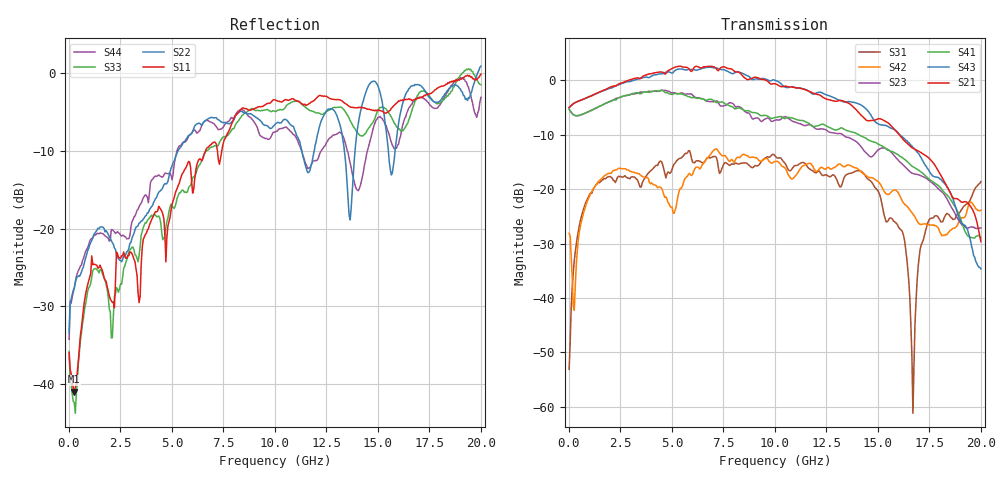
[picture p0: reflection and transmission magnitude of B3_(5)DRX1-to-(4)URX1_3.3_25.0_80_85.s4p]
!Agilent Technologies,N5225A,MY51451112,A.09.50.13
!Agilent N5225A: A.09.50.13
!Date: Sunday, March 12, 2017 05:21:35
!Correction: S11(Full 4 Port(1,2,3,4))
!S12(Full 4 Port(1,2,3,4))
!S13(Full 4 Port(1,2,3,4))
!S14(Full 4 Port(1,2,3,4))
!S21(Full 4 Port(1,2,3,4))
!S22(Full 4 Port(1,2,3,4))
!S23(Full 4 Port(1,2,3,4))
!S24(Full 4 Port(1,2,3,4))
!S31(Full 4 Port(1,2,3,4))
!S32(Full 4 Port(1,2,3,4))
!S33(Full 4 Port(1,2,3,4))
!S34(Full 4 Port(1,2,3,4))
!S41(Full 4 Port(1,2,3,4))
!S42(Full 4 Port(1,2,3,4))
!S43(Full 4 Port(1,2,3,4))
!S44(Full 4 Port(1,2,3,4))
!S4P File: Measurements: <S11,S12,S13,S14>,
!<S21,S22,S23,S24>,
!<S31,S32,S33,S34>,
!<S41,S42,S43,S44>:
# Hz S  dB  R 50
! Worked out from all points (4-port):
!   401 points, 10 MHz to 20 GHz, reference 50 ohm
!   strongest paths, dB at 10 MHz, 5.008 GHz, 10.01 GHz, 15 GHz, 20 GHz:
!     S21: -5.0, 2.2, -0.7, -7.1, -29.6
!     S43: -5.0, 1.3, 0.0, -8.0, -34.7
!     S41: -5.3, -2.6, -6.9, -11.7, -28.9
!     S23: -5.3, -2.3, -7.3, -12.8, -27.1
!     S42: -28.1, -23.3, -14.9, -18.6, -23.9
!     S31: -53.1, -16.4, -13.9, -20.3, -18.6
!   lowest |S11| = -40.9 dB at 259.9 MHz (marker M1), VSWR 1.02, Z = 50.3 - j0.86 ohm
!   |S11| at or under -10 dB: start of sweep to 6.636 GHz; 7.207 GHz to 7.422 GHz (214.9 MHz wide, 2.94 % of centre)
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1e7  -35.94 -38.5  -66.81 145.0  -53.30 11.9  -77.60 160.5
     -5.02 1.4  -33.41 38.9  -5.33 -179.9  -28.03 37.7
     -53.11 17.5  -71.79 97.3  -35.75 -45.8  -64.70 94.1
     -5.33 -179.9  -28.10 38.0  -5.00 1.6  -34.23 44.1
2.59875e8  -40.92 -72.0  -49.86 56.0  -33.16 94.7  -50.74 54.6
           -4.21 -2.2  -27.63 -131.8  -6.43 169.7  -41.81 -161.8
           -33.21 95.3  -49.91 57.8  -42.28 -78.8  -50.44 56.6
           -6.43 168.9  -42.26 -171.1  -4.19 -3.0  -27.67 -137.7
5.157425e9  -15.53 88.5  -37.75 12.0  -15.42 29.2  -39.42 -18.5
            2.41 173.7  -10.99 143.9  -2.36 -27.1  -24.24 57.7
            -15.21 27.6  -37.57 1.9  -17.15 103.9  -38.59 -54.3
            -2.43 -42.8  -23.82 59.0  1.80 163.8  -11.01 122.8
8.255875e9  -5.04 37.1  -39.67 -109.5  -15.53 -0.5  -36.36 -138.8
            1.46 21.1  -5.06 80.8  -4.85 -161.1  -13.85 47.6
            -15.39 -1.1  -32.44 -115.7  -6.08 58.7  -31.73 -151.8
            -5.06 175.9  -14.21 50.2  1.48 8.3  -4.87 45.5
1.215392e10  -2.93 -17.6  -33.33 -149.2  -16.32 -21.1  -34.60 170.5
             -2.69 -145.1  -7.01 66.9  -8.99 37.4  -16.04 40.2
             -16.68 -20.3  -34.12 -142.1  -5.20 -3.6  -33.11 175.4
             -8.29 1.3  -16.29 42.9  -2.19 -169.3  -10.57 -6.3
1.670165e10  -3.53 -75.7  -34.84 118.1  -50.91 9.9  -36.57 86.3
             -12.49 13.7  -1.63 65.9  -17.14 170.5  -24.78 57.1
             -61.18 55.9  -33.11 122.1  -4.42 -82.3  -33.10 84.0
             -15.88 118.3  -24.62 57.3  -12.32 -36.2  -3.70 -61.2
2e10  -0.18 -114.1  -32.97 63.0  -18.65 121.4  -35.51 21.5
      -29.64 -142.1  0.84 17.1  -27.12 34.9  -23.90 101.9
      -18.62 121.4  -34.02 40.5  -1.54 -87.6  -35.24 -8.0
      -28.91 -9.1  -23.90 102.7  -34.67 -168.2  -3.17 -136.4
